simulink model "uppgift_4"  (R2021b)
settings: Solver=VariableStepAuto  StartTime=0.0  StopTime=10.0  RelTol=1e-3
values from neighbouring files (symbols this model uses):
  AFs = 14.6    [Lektion_2.m]
  eta_vol = 0.8    [Lektion_2.m]
  m_dot_fi_start = m_dot_a_start/AFs    (= 0.000821917808219)    [Lektion_2.m]
  n_cyl = 4    [Lektion_2.m]
  N_init = 3000/60    (= 50)    [Lektion_2.m]
  n_r = 2    [Lektion_2.m]
  p_im_end = 70*1e3    (= 70000)    [Lektion_2.m]
  p_im_init = 40*1e3    (= 40000)    [Lektion_2.m]
  R = 280    [Lektion_2.m]
  T_i = 320    [Lektion_2.m]
  V_d = 0.55/1e3    (= 0.00055)    [Lektion_2.m]

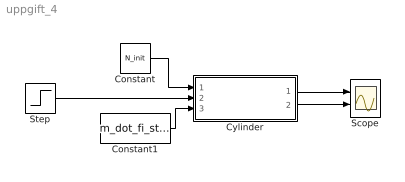
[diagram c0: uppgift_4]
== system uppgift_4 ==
  Constant : Constant  Value=N_init
  Constant1 : Constant  Value=m_dot_fi_start
  Cylinder : Subsystem
  Scope : Scope  NumInputPorts=2
  Step : Step  Before=p_im_init  After=p_im_end  SampleTime=0
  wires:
  Constant/1 -> Cylinder/1(N [rps])
  Constant1/1 -> Cylinder/3(m_fi [kg/s])
  Step/1 -> Cylinder/2(p_im [Pa])
  Cylinder/1(m_ac [kg/s]) -> Scope/1
  Cylinder/2(lambda_c [-]) -> Scope/2

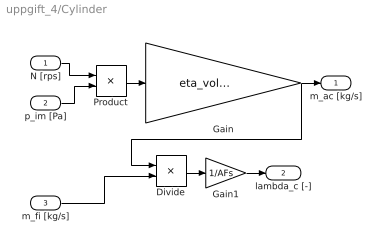
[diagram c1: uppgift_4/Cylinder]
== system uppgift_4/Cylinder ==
  N [rps] : Inport
  p_im [Pa] : Inport  Port=2
  m_fi [kg/s] : Inport  Port=3
  Divide : Product  Inputs=*/
  Gain : Gain  Gain=eta_vol*V_d*n_cyl/(n_r*R*T_i)
  Gain1 : Gain  Gain=1/AFs
  Product : Product
  m_ac [kg/s] : Outport
  lambda_c [-] : Outport  Port=2
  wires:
  N [rps]/1 -> Product/1
  p_im [Pa]/1 -> Product/2
  Product/1 -> Gain/1
  Gain/1 -> Divide/1, m_ac [kg/s]/1
  m_fi [kg/s]/1 -> Divide/2
  Divide/1 -> Gain1/1
  Gain1/1 -> lambda_c [-]/1
